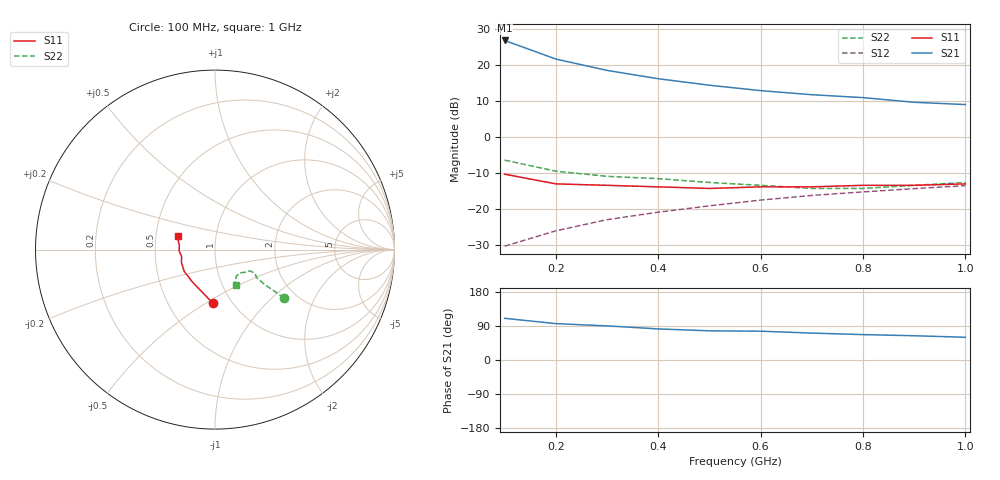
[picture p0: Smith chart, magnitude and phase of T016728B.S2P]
!AT-01672
!S-PARAMETERS at Vce=8V  Ic=60mA.  LAST UPDATED 07-21-92
!OBSOLETED Feb 1994 - nearest replacement: AT-42070
# ghz s ma r 50
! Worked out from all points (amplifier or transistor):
!   10 points, 100 MHz to 1 GHz, reference 50 ohm
!   highest |S21| = 26.7 dB at 100 MHz (marker M1)
!   |S21| within 3 dB of that: start of sweep to 158.1 MHz
!   unconditionally stable (mu >= 1): 322.4 MHz to end of sweep
!   at 200 MHz: K = 0.95, MSG = 23.9 dB, |S12| = -26.2 dB
!   at 600 MHz: K = 1.05, MAG = 13.8 dB, |S12| = -17.7 dB
!   at 1 GHz: K = 1.02, MAG = 10.3 dB, |S12| = -13.6 dB
0.1  0.3 -92.0  21.6 110.0  0.03 73.0  0.47 -35.0
0.2  0.22 -125.0  11.92 96.0  0.049 76.0  0.33 -35.0
0.3  0.21 -145.0  8.29 90.0  0.07 75.0  0.28 -34.0
0.4  0.2 -159.0  6.35 82.0  0.089 72.0  0.26 -31.0
0.5  0.19 -169.0  5.16 77.0  0.109 70.0  0.23 -31.0
0.6  0.2 -178.0  4.34 76.0  0.131 72.0  0.21 -37.0
0.7  0.2 173.0  3.81 71.0  0.152 68.0  0.19 -43.0
0.8  0.21 167.0  3.47 67.0  0.17 66.0  0.19 -51.0
0.9  0.21 165.0  2.99 64.0  0.189 67.0  0.21 -58.0
1  0.22 160.0  2.78 60.0  0.208 64.0  0.23 -60.0
